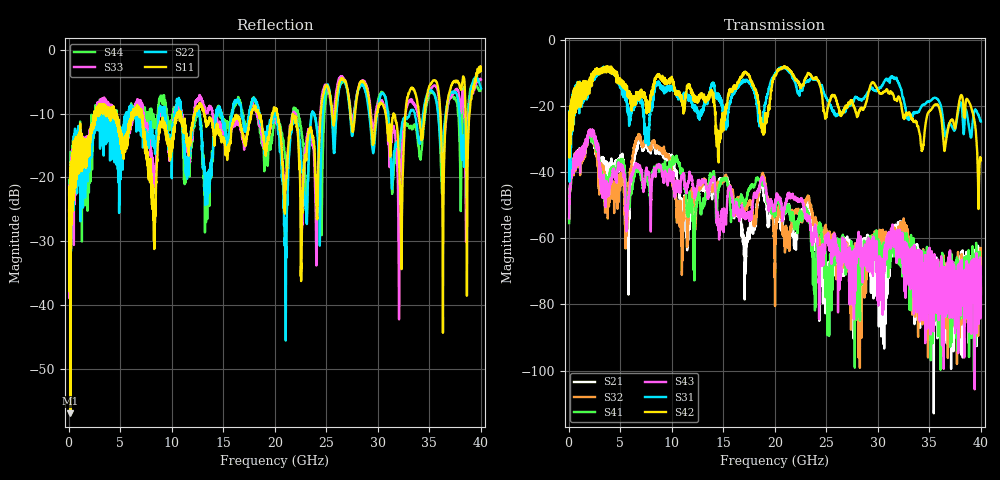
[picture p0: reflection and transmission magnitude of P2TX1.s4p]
!Agilent Technologies,N5245A,MY49151084,A.09.20.08
!Agilent N5245A: A.09.20.08
!Date: Thursday, March 01, 2012 14:27:59
!Correction: S11(Full 4 Port(1,2,3,4))
!S12(Full 4 Port(1,2,3,4))
!S13(Full 4 Port(1,2,3,4))
!S14(Full 4 Port(1,2,3,4))
!S21(Full 4 Port(1,2,3,4))
!S22(Full 4 Port(1,2,3,4))
!S23(Full 4 Port(1,2,3,4))
!S24(Full 4 Port(1,2,3,4))
!S31(Full 4 Port(1,2,3,4))
!S32(Full 4 Port(1,2,3,4))
!S33(Full 4 Port(1,2,3,4))
!S34(Full 4 Port(1,2,3,4))
!S41(Full 4 Port(1,2,3,4))
!S42(Full 4 Port(1,2,3,4))
!S43(Full 4 Port(1,2,3,4))
!S44(Full 4 Port(1,2,3,4))
!S4P File: Measurements: <S11,S12,S13,S14>,
!<S21,S22,S23,S24>,
!<S31,S32,S33,S34>,
!<S41,S42,S43,S44>:
# Hz S  dB  R 50
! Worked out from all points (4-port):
!   3996 points, 50 MHz to 40 GHz, reference 50 ohm
!   strongest paths, dB at 50 MHz, 10.04 GHz, 20.03 GHz, 30.02 GHz, 40 GHz:
!     S42: -24.4, -12.2, -10.8, -15.3, -36.4
!     S31: -27.2, -14.2, -10.1, -14.9, -24.7
!     S43: -54.0, -40.5, -49.1, -75.1, -76.9
!     S41: -55.4, -36.7, -52.2, -63.1, -71.6
!     S32: -54.6, -43.1, -80.5, -62.5, -75.0
!     S21: -54.0, -36.7, -56.2, -66.8, -80.1
!   lowest |S11| = -57.0 dB at 180 MHz (marker M1), VSWR 1.00, Z = 50.1 - j0.0734 ohm
!   |S11| at or under -10 dB: 7.102 GHz to 10.54 GHz (3.435 GHz wide, 38.9 % of centre); 13.15 GHz to 17.72 GHz (4.573 GHz wide, 29.6 % of centre); 20.22 GHz to 24.46 GHz (4.237 GHz wide, 19 % of centre)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
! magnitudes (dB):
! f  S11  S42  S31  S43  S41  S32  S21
! 50 MHz  -25.2  -24.4  -27.2  -54.0  -55.4  -54.6  -54.0
! 180 MHz  -57.0  -26.8  -29.3  -42.9  -42.9  -43.3  -43.3
! 5.61 GHz  -14.0  -14.5  -17.8  -57.9  -48.6  -54.4  -48.1
! 6.78 GHz  -10.2  -18.2  -17.0  -38.1  -39.4  -28.4  -30.4
! 17.99 GHz  -8.8  -14.6  -15.4  -46.5  -44.5  -54.9  -56.0
! 21.04 GHz  -21.8  -8.3  -8.7  -49.4  -50.5  -58.6  -51.7
! 40 GHz  -3.3  -36.4  -24.7  -76.9  -71.6  -75.0  -80.1
